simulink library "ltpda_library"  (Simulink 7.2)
settings: Solver=ode45  SolverMode=SingleTasking  StartTime=0.0  StopTime=10.0  RelTol=1e-3
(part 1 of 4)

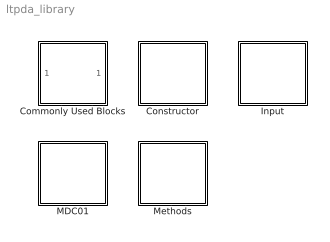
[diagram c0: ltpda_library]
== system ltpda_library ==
  Commonly Used Blocks : Subsystem
  Constructor : Subsystem  Tag=subsystem  AncestorBlock=libraryBase/SubSystName
  Input : Subsystem
  MDC01 : Subsystem  Tag=subsystem  AncestorBlock=libraryBase/SubSystName
  Methods : Subsystem  Tag=subsystem  AncestorBlock=libraryBase/SubSystName

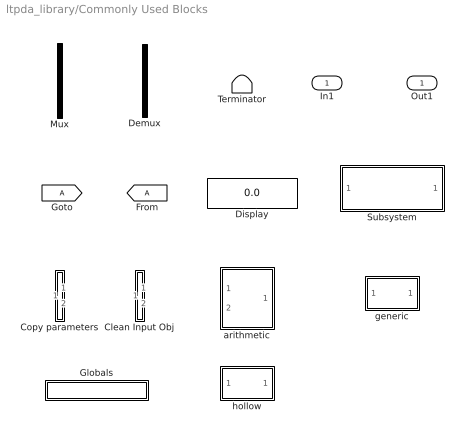
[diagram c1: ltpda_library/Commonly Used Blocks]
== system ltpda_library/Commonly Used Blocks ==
  In1 : Inport  OutDataType=sfix(16)  OutScaling=2^0
  Clean Input Obj : Subsystem
  Copy parameters : Subsystem
  Demux : Demux  Tag=demux  Outputs=2
  Display : Display
  Globals : Subsystem  Tag=globals
  Mux : Mux  Tag=mux  Inputs=2
  Subsystem : Subsystem
  Terminator : Terminator
  arithmetic : Subsystem  Tag=arithmetic
  generic : Subsystem  Tag=function
  hollow : Subsystem  Tag=method ao
  Out1 : Outport  OutDataType=sfix(16)  OutScaling=2^0

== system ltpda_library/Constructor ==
  ltpda_getAOsInTimeSpan : Subsystem  Tag=function  AncestorBlock=libraryBase/function

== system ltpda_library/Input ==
  Constructor : Subsystem  Tag=method ltpda_gui
  Object from list : Subsystem  Tag=input

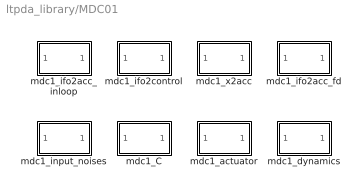
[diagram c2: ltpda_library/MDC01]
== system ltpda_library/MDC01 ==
  mdc1_C : Subsystem  Tag=function  AncestorBlock=libraryBase/function
  mdc1_actuator : Subsystem  Tag=function  AncestorBlock=libraryBase/function
  mdc1_dynamics : Subsystem  Tag=function  AncestorBlock=libraryBase/function
  mdc1_ifo2acc_fd : Subsystem  Tag=function  AncestorBlock=libraryBase/function
  mdc1_ifo2acc_inloop : Subsystem  Tag=function  AncestorBlock=libraryBase/function
  mdc1_ifo2control : Subsystem  Tag=function  AncestorBlock=libraryBase/function
  mdc1_input_noises : Subsystem  Tag=function  AncestorBlock=libraryBase/function
  mdc1_x2acc : Subsystem  Tag=function  AncestorBlock=libraryBase/function

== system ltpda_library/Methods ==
  ao : Subsystem  Tag=subsystem  AncestorBlock=libraryBase/SubSystName

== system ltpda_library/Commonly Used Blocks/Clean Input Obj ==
  In1 : Inport  OutDataType=sfix(16)  OutScaling=2^0
  In2 : Inport  Port=2  OutDataType=sfix(16)  OutScaling=2^0
  cleaninput : M-S-Function  FunctionName=g_cleaninput
  Out1 : Outport  OutDataType=sfix(16)  OutScaling=2^0
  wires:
  In2/1 -> cleaninput/2
  In1/1 -> cleaninput/1
  cleaninput/1 -> Out1/1

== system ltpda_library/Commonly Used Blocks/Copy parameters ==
  In1 : Inport  OutDataType=sfix(16)  OutScaling=2^0
  In2 : Inport  Port=2  OutDataType=sfix(16)  OutScaling=2^0
  copyparam : M-S-Function  FunctionName=g_copyparams
  Out1 : Outport  OutDataType=sfix(16)  OutScaling=2^0
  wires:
  copyparam/1 -> Out1/1
  In1/1 -> copyparam/1
  In2/1 -> copyparam/2

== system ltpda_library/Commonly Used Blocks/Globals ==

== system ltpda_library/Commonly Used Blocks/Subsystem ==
  In1 : Inport  OutDataType=sfix(16)  OutScaling=2^0
  Out1 : Outport  OutDataType=sfix(16)  OutScaling=2^0

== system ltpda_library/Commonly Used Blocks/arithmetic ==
  alpha : Inport  Tag=1  OutDataType=sfix(16)  OutScaling=2^0
  beta : Inport  Tag=2  Port=2  OutDataType=sfix(16)  OutScaling=2^0
  Mux : Mux  Tag=mux  Inputs=2
  arithmetic_func : M-S-Function  Tag=arithmetic  FunctionName=ltpdasim
  Out1 : Outport  OutDataType=sfix(16)  OutScaling=2^0
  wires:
  arithmetic_func/1 -> Out1/1
  Mux/1 -> arithmetic_func/1
  alpha/1 -> Mux/1
  beta/1 -> Mux/2

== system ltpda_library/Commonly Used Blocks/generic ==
  In1 : Inport  OutDataType=sfix(16)  OutScaling=2^0
  generic : M-S-Function  Tag=generic  FunctionName=ltpdasim
  Out1 : Outport  OutDataType=sfix(16)  OutScaling=2^0
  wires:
  generic/1 -> Out1/1
  In1/1 -> generic/1

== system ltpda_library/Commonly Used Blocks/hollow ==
  In1 : Inport  OutDataType=sfix(16)  OutScaling=2^0
  hollow : M-S-Function  FunctionName=ltpdasim
  Out1 : Outport  OutDataType=sfix(16)  OutScaling=2^0
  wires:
  In1/1 -> hollow/1
  hollow/1 -> Out1/1

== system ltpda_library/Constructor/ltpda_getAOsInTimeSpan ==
  In1 : Inport  OutDataType=sfix(16)  OutScaling=2^0
  ltpda_getAOsInTimeSpan : M-S-Function  Tag=ltpda_getAOsInTimeSpan  FunctionName=ltpdasim
  Out1 : Outport  OutDataType=sfix(16)  OutScaling=2^0
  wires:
  In1/1 -> ltpda_getAOsInTimeSpan/1
  ltpda_getAOsInTimeSpan/1 -> Out1/1

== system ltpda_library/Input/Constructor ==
  Ground : Ground
  g_constructor : M-S-Function  Tag=g_constructor  FunctionName=ltpdasim
  Out1 : Outport  OutDataType=sfix(16)  OutScaling=2^0
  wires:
  g_constructor/1 -> Out1/1
  Ground/1 -> g_constructor/1

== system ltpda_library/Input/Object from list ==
  Input : Constant  Value=0  OutDataType=sfix(16)  OutScaling=2^0
  Input AO : Outport  OutDataType=sfix(16)  OutScaling=2^0
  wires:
  Input/1 -> Input AO/1

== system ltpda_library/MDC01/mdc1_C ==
  In1 : Inport  OutDataType=sfix(16)  OutScaling=2^0
  ltpda_mdc1_C : M-S-Function  Tag=ltpda_mdc1_C  FunctionName=ltpdasim
  Out1 : Outport  OutDataType=sfix(16)  OutScaling=2^0
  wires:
  In1/1 -> ltpda_mdc1_C/1
  ltpda_mdc1_C/1 -> Out1/1

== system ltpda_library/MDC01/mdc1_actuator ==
  In1 : Inport  OutDataType=sfix(16)  OutScaling=2^0
  ltpda_mdc1_actuator : M-S-Function  Tag=ltpda_mdc1_actuator  FunctionName=ltpdasim
  Out1 : Outport  OutDataType=sfix(16)  OutScaling=2^0
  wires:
  In1/1 -> ltpda_mdc1_actuator/1
  ltpda_mdc1_actuator/1 -> Out1/1

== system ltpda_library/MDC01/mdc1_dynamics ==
  In1 : Inport  OutDataType=sfix(16)  OutScaling=2^0
  ltpda_mdc1_dynamics : M-S-Function  Tag=ltpda_mdc1_dynamics  FunctionName=ltpdasim
  Out1 : Outport  OutDataType=sfix(16)  OutScaling=2^0
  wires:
  In1/1 -> ltpda_mdc1_dynamics/1
  ltpda_mdc1_dynamics/1 -> Out1/1

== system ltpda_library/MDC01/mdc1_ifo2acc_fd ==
  In1 : Inport  OutDataType=sfix(16)  OutScaling=2^0
  ltpda_mdc1_ifo2acc_fd : M-S-Function  Tag=ltpda_mdc1_ifo2acc_fd  FunctionName=ltpdasim
  Out1 : Outport  OutDataType=sfix(16)  OutScaling=2^0
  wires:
  In1/1 -> ltpda_mdc1_ifo2acc_fd/1
  ltpda_mdc1_ifo2acc_fd/1 -> Out1/1

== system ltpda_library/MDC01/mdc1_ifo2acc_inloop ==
  In1 : Inport  OutDataType=sfix(16)  OutScaling=2^0
  ltpda_mdc1_ifo2acc_inloop : M-S-Function  Tag=ltpda_mdc1_ifo2acc_inloop  FunctionName=ltpdasim
  Out1 : Outport  OutDataType=sfix(16)  OutScaling=2^0
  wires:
  In1/1 -> ltpda_mdc1_ifo2acc_inloop/1
  ltpda_mdc1_ifo2acc_inloop/1 -> Out1/1

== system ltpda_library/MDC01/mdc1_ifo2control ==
  In1 : Inport  OutDataType=sfix(16)  OutScaling=2^0
  ltpda_mdc1_ifo2control : M-S-Function  Tag=ltpda_mdc1_ifo2control  FunctionName=ltpdasim
  Out1 : Outport  OutDataType=sfix(16)  OutScaling=2^0
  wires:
  In1/1 -> ltpda_mdc1_ifo2control/1
  ltpda_mdc1_ifo2control/1 -> Out1/1

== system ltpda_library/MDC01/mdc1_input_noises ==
  In1 : Inport  OutDataType=sfix(16)  OutScaling=2^0
  ltpda_mdc1_input_noises : M-S-Function  Tag=ltpda_mdc1_input_noises  FunctionName=ltpdasim
  Out1 : Outport  OutDataType=sfix(16)  OutScaling=2^0
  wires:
  In1/1 -> ltpda_mdc1_input_noises/1
  ltpda_mdc1_input_noises/1 -> Out1/1

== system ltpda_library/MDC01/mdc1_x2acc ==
  In1 : Inport  OutDataType=sfix(16)  OutScaling=2^0
  ltpda_mdc1_x2acc : M-S-Function  Tag=ltpda_mdc1_x2acc  FunctionName=ltpdasim
  Out1 : Outport  OutDataType=sfix(16)  OutScaling=2^0
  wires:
  In1/1 -> ltpda_mdc1_x2acc/1
  ltpda_mdc1_x2acc/1 -> Out1/1

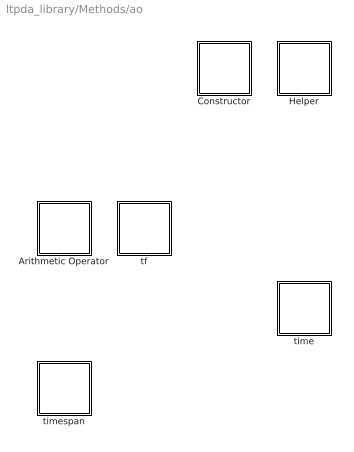
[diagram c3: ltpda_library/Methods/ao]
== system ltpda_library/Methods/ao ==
  Arithmetic Operator : Subsystem  Tag=subsystem  AncestorBlock=libraryBase/SubSystName
  Constructor : Subsystem  Tag=subsystem  AncestorBlock=libraryBase/SubSystName
  Helper : Subsystem  Tag=subsystem  AncestorBlock=libraryBase/SubSystName
  time : Subsystem  Tag=subsystem  AncestorBlock=libraryBase/SubSystName
  tf : Subsystem  Tag=subsystem  AncestorBlock=libraryBase/SubSystName
  time : Subsystem  Tag=subsystem  AncestorBlock=libraryBase/SubSystName
  timespan : Subsystem  Tag=subsystem  AncestorBlock=libraryBase/SubSystName

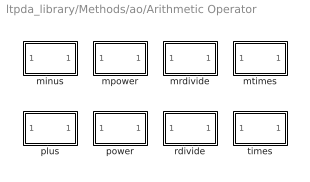
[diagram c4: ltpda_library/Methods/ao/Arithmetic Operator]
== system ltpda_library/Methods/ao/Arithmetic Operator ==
  minus : Subsystem  Tag=method ao  AncestorBlock=libraryBase/function
  mpower : Subsystem  Tag=method ao  AncestorBlock=libraryBase/function
  mrdivide : Subsystem  Tag=method ao  AncestorBlock=libraryBase/function
  mtimes : Subsystem  Tag=method ao  AncestorBlock=libraryBase/function
  plus : Subsystem  Tag=method ao  AncestorBlock=libraryBase/function
  power : Subsystem  Tag=method ao  AncestorBlock=libraryBase/function
  rdivide : Subsystem  Tag=method ao  AncestorBlock=libraryBase/function
  times : Subsystem  Tag=method ao  AncestorBlock=libraryBase/function

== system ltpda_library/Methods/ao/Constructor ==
  ao : Subsystem  Tag=method ao  AncestorBlock=libraryBase/constructor  AncestorBlock=libraryBase/constructor
  rebuild : Subsystem  Tag=method ao  AncestorBlock=libraryBase/constructor

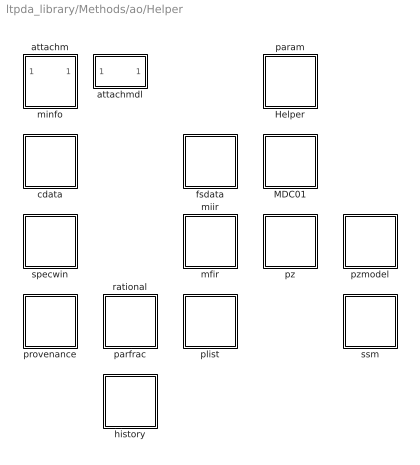
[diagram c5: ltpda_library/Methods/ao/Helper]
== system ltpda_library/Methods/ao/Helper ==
  attachm : Subsystem  Tag=method ao  AncestorBlock=libraryBase/function  AncestorBlock=libraryBase/constructor
  attachmdl : Subsystem  Tag=method ao  AncestorBlock=libraryBase/function
  Helper : Subsystem  Tag=subsystem  AncestorBlock=libraryBase/SubSystName
  MDC01 : Subsystem  Tag=subsystem  AncestorBlock=libraryBase/SubSystName
  cdata : Subsystem  Tag=subsystem  AncestorBlock=libraryBase/SubSystName
  fsdata : Subsystem  Tag=subsystem  AncestorBlock=libraryBase/SubSystName
  history : Subsystem  Tag=subsystem  AncestorBlock=libraryBase/SubSystName
  mfir : Subsystem  Tag=subsystem  AncestorBlock=libraryBase/SubSystName
  miir : Subsystem  Tag=subsystem  AncestorBlock=libraryBase/SubSystName
  miir : Subsystem  Tag=subsystem  AncestorBlock=libraryBase/SubSystName
  minfo : Subsystem  Tag=subsystem  AncestorBlock=libraryBase/SubSystName
  param : Subsystem  Tag=subsystem  AncestorBlock=libraryBase/SubSystName
  plist : Subsystem  Tag=subsystem  AncestorBlock=libraryBase/SubSystName
  provenance : Subsystem  Tag=subsystem  AncestorBlock=libraryBase/SubSystName
  pz : Subsystem  Tag=subsystem  AncestorBlock=libraryBase/SubSystName
  pzmodel : Subsystem  Tag=subsystem  AncestorBlock=libraryBase/SubSystName
  specwin : Subsystem  Tag=subsystem  AncestorBlock=libraryBase/SubSystName
  cdata : Subsystem  Tag=subsystem  AncestorBlock=libraryBase/SubSystName
  fsdata : Subsystem  Tag=subsystem  AncestorBlock=libraryBase/SubSystName
  history : Subsystem  Tag=subsystem  AncestorBlock=libraryBase/SubSystName
  mfir : Subsystem  Tag=subsystem  AncestorBlock=libraryBase/SubSystName
  miir : Subsystem  Tag=subsystem  AncestorBlock=libraryBase/SubSystName
  minfo : Subsystem  Tag=subsystem  AncestorBlock=libraryBase/SubSystName
  param : Subsystem  Tag=subsystem  AncestorBlock=libraryBase/SubSystName
  parfrac : Subsystem  Tag=subsystem  AncestorBlock=libraryBase/SubSystName
  plist : Subsystem  Tag=subsystem  AncestorBlock=libraryBase/SubSystName
  provenance : Subsystem  Tag=subsystem  AncestorBlock=libraryBase/SubSystName
  pz : Subsystem  Tag=subsystem  AncestorBlock=libraryBase/SubSystName
  pzmodel : Subsystem  Tag=subsystem  AncestorBlock=libraryBase/SubSystName
  rational : Subsystem  Tag=subsystem  AncestorBlock=libraryBase/SubSystName
  specwin : Subsystem  Tag=subsystem  AncestorBlock=libraryBase/SubSystName
  ssm : Subsystem  Tag=subsystem  AncestorBlock=libraryBase/SubSystName
  ssm : Subsystem  Tag=subsystem  AncestorBlock=libraryBase/SubSystName

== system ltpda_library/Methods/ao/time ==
  Arithmetic Operator : Subsystem  Tag=subsystem  AncestorBlock=libraryBase/SubSystName

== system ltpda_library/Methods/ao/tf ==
  Constructor : Subsystem  Tag=subsystem  AncestorBlock=libraryBase/SubSystName
  Helper : Subsystem  Tag=subsystem  AncestorBlock=libraryBase/SubSystName
  Output : Subsystem  Tag=subsystem  AncestorBlock=libraryBase/SubSystName
  Relational Operator : Subsystem  Tag=subsystem  AncestorBlock=libraryBase/SubSystName

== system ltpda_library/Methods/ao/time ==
  Arithmetic Operator : Subsystem  Tag=subsystem  AncestorBlock=libraryBase/SubSystName
  Constructor : Subsystem  Tag=subsystem  AncestorBlock=libraryBase/SubSystName
  Helper : Subsystem  Tag=subsystem  AncestorBlock=libraryBase/SubSystName
  Output : Subsystem  Tag=subsystem  AncestorBlock=libraryBase/SubSystName
  Relational Operator : Subsystem  Tag=subsystem  AncestorBlock=libraryBase/SubSystName
  Relational Operator : Subsystem  Tag=subsystem  AncestorBlock=libraryBase/SubSystName

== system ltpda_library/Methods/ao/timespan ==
  Constructor : Subsystem  Tag=subsystem  AncestorBlock=libraryBase/SubSystName
  Helper : Subsystem  Tag=subsystem  AncestorBlock=libraryBase/SubSystName

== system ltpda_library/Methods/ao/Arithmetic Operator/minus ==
  In1 : Inport  OutDataType=sfix(16)  OutScaling=2^0
  minus : M-S-Function  Tag=minus  FunctionName=ltpdasim
  Out1 : Outport  OutDataType=sfix(16)  OutScaling=2^0
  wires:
  In1/1 -> minus/1
  minus/1 -> Out1/1

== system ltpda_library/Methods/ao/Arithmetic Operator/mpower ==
  In1 : Inport  OutDataType=sfix(16)  OutScaling=2^0
  mpower : M-S-Function  Tag=mpower  FunctionName=ltpdasim
  Out1 : Outport  OutDataType=sfix(16)  OutScaling=2^0
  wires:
  In1/1 -> mpower/1
  mpower/1 -> Out1/1

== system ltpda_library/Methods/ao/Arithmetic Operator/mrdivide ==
  In1 : Inport  OutDataType=sfix(16)  OutScaling=2^0
  mrdivide : M-S-Function  Tag=mrdivide  FunctionName=ltpdasim
  Out1 : Outport  OutDataType=sfix(16)  OutScaling=2^0
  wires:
  In1/1 -> mrdivide/1
  mrdivide/1 -> Out1/1

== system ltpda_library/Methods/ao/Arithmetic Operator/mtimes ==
  In1 : Inport  OutDataType=sfix(16)  OutScaling=2^0
  mtimes : M-S-Function  Tag=mtimes  FunctionName=ltpdasim
  Out1 : Outport  OutDataType=sfix(16)  OutScaling=2^0
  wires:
  In1/1 -> mtimes/1
  mtimes/1 -> Out1/1

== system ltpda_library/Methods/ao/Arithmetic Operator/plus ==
  In1 : Inport  OutDataType=sfix(16)  OutScaling=2^0
  plus : M-S-Function  Tag=plus  FunctionName=ltpdasim
  Out1 : Outport  OutDataType=sfix(16)  OutScaling=2^0
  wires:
  In1/1 -> plus/1
  plus/1 -> Out1/1

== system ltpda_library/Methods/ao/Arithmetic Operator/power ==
  In1 : Inport  OutDataType=sfix(16)  OutScaling=2^0
  power : M-S-Function  Tag=power  FunctionName=ltpdasim
  Out1 : Outport  OutDataType=sfix(16)  OutScaling=2^0
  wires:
  In1/1 -> power/1
  power/1 -> Out1/1

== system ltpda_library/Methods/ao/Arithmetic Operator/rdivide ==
  In1 : Inport  OutDataType=sfix(16)  OutScaling=2^0
  rdivide : M-S-Function  Tag=rdivide  FunctionName=ltpdasim
  Out1 : Outport  OutDataType=sfix(16)  OutScaling=2^0
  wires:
  In1/1 -> rdivide/1
  rdivide/1 -> Out1/1

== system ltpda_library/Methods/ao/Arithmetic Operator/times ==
  In1 : Inport  OutDataType=sfix(16)  OutScaling=2^0
  times : M-S-Function  Tag=times  FunctionName=ltpdasim
  Out1 : Outport  OutDataType=sfix(16)  OutScaling=2^0
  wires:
  In1/1 -> times/1
  times/1 -> Out1/1

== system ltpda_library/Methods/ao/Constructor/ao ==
  Ground : Ground
  ao : M-S-Function  Tag=ao  FunctionName=ltpdasim
  Out1 : Outport  OutDataType=sfix(16)  OutScaling=2^0
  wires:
  Ground/1 -> ao/1
  ao/1 -> Out1/1

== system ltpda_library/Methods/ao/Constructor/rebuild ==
  Ground : Ground
  rebuild : M-S-Function  Tag=rebuild  FunctionName=ltpdasim
  Out1 : Outport  OutDataType=sfix(16)  OutScaling=2^0
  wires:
  Ground/1 -> rebuild/1
  rebuild/1 -> Out1/1

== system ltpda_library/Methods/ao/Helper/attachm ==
  In1 : Inport  OutDataType=sfix(16)  OutScaling=2^0
  rebuild : M-S-Function  Tag=attachm  Tag=rebuild  FunctionName=ltpdasim
  Out1 : Outport  OutDataType=sfix(16)  OutScaling=2^0
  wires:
  In1/1 -> rebuild/1
  rebuild/1 -> Out1/1

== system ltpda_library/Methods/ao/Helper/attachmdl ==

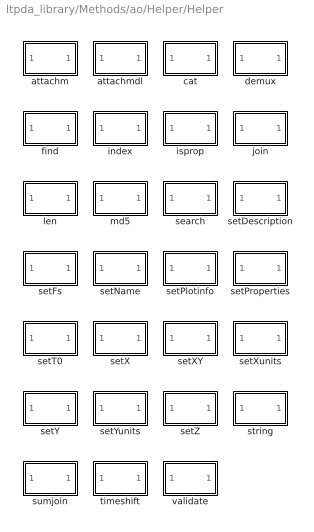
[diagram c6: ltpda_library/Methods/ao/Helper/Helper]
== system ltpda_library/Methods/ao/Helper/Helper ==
  attachm : Subsystem  Tag=method ao  AncestorBlock=libraryBase/function
  attachmdl : Subsystem  Tag=method ao  AncestorBlock=libraryBase/function
  cat : Subsystem  Tag=method ao  AncestorBlock=libraryBase/function
  demux : Subsystem  Tag=method ao  AncestorBlock=libraryBase/function
  find : Subsystem  Tag=method ao  AncestorBlock=libraryBase/function
  index : Subsystem  Tag=method ao  AncestorBlock=libraryBase/function
  isprop : Subsystem  Tag=method ao  AncestorBlock=libraryBase/function
  join : Subsystem  Tag=method ao  AncestorBlock=libraryBase/function
  len : Subsystem  Tag=method ao  AncestorBlock=libraryBase/function
  md5 : Subsystem  Tag=method ao  AncestorBlock=libraryBase/function
  search : Subsystem  Tag=method ao  AncestorBlock=libraryBase/function
  setDescription : Subsystem  Tag=method ao  AncestorBlock=libraryBase/function
  setFs : Subsystem  Tag=method ao  AncestorBlock=libraryBase/function
  setName : Subsystem  Tag=method ao  AncestorBlock=libraryBase/function
  setPlotinfo : Subsystem  Tag=method ao  AncestorBlock=libraryBase/function
  setProperties : Subsystem  Tag=method ao  AncestorBlock=libraryBase/function
  setPlotinfo : Subsystem  Tag=method ao  AncestorBlock=libraryBase/function
  setProperties : Subsystem  Tag=method ao  AncestorBlock=libraryBase/function
  setT0 : Subsystem  Tag=method ao  AncestorBlock=libraryBase/function
  setX : Subsystem  Tag=method ao  AncestorBlock=libraryBase/function
  setXY : Subsystem  Tag=method ao  AncestorBlock=libraryBase/function
  setXunits : Subsystem  Tag=method ao  AncestorBlock=libraryBase/function
  setY : Subsystem  Tag=method ao  AncestorBlock=libraryBase/function
  setYunits : Subsystem  Tag=method ao  AncestorBlock=libraryBase/function
  setZ : Subsystem  Tag=method ao  AncestorBlock=libraryBase/function
  string : Subsystem  Tag=method ao  AncestorBlock=libraryBase/function
  sumjoin : Subsystem  Tag=method ao  AncestorBlock=libraryBase/function
  sumjoin : Subsystem  Tag=method ao  AncestorBlock=libraryBase/function
  timeshift : Subsystem  Tag=method ao  AncestorBlock=libraryBase/function
  validate : Subsystem  Tag=method ao  AncestorBlock=libraryBase/function

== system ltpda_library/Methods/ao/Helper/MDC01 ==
  mdc1_ifo2acc_fd : Subsystem  Tag=method ao  AncestorBlock=libraryBase/function
  mdc1_ifo2acc_inloop : Subsystem  Tag=method ao  AncestorBlock=libraryBase/function
  mdc1_ifo2control : Subsystem  Tag=method ao  AncestorBlock=libraryBase/function

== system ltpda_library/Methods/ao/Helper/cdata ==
  Constructor : Subsystem  Tag=subsystem  AncestorBlock=libraryBase/SubSystName
  Helper : Subsystem  Tag=subsystem  AncestorBlock=libraryBase/SubSystName
  Output : Subsystem  Tag=subsystem  AncestorBlock=libraryBase/SubSystName
  Relational Operator : Subsystem  Tag=subsystem  AncestorBlock=libraryBase/SubSystName

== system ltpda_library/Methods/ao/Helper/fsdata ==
  Constructor : Subsystem  Tag=subsystem  AncestorBlock=libraryBase/SubSystName
  Helper : Subsystem  Tag=subsystem  AncestorBlock=libraryBase/SubSystName
  Output : Subsystem  Tag=subsystem  AncestorBlock=libraryBase/SubSystName
  Relational Operator : Subsystem  Tag=subsystem  AncestorBlock=libraryBase/SubSystName

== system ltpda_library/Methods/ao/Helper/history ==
  Constructor : Subsystem  Tag=subsystem  AncestorBlock=libraryBase/SubSystName
  Helper : Subsystem  Tag=subsystem  AncestorBlock=libraryBase/SubSystName
  Output : Subsystem  Tag=subsystem  AncestorBlock=libraryBase/SubSystName
  Relational Operator : Subsystem  Tag=subsystem  AncestorBlock=libraryBase/SubSystName

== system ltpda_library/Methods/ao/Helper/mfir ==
  Constructor : Subsystem  Tag=subsystem  AncestorBlock=libraryBase/SubSystName
  Helper : Subsystem  Tag=subsystem  AncestorBlock=libraryBase/SubSystName
  Output : Subsystem  Tag=subsystem  AncestorBlock=libraryBase/SubSystName
  Relational Operator : Subsystem  Tag=subsystem  AncestorBlock=libraryBase/SubSystName
  Signal Processing : Subsystem  Tag=subsystem  AncestorBlock=libraryBase/SubSystName
  Statespace : Subsystem  Tag=subsystem  AncestorBlock=libraryBase/SubSystName

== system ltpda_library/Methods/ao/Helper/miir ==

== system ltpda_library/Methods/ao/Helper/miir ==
  Constructor : Subsystem  Tag=subsystem  AncestorBlock=libraryBase/SubSystName
  Helper : Subsystem  Tag=subsystem  AncestorBlock=libraryBase/SubSystName
  Output : Subsystem  Tag=subsystem  AncestorBlock=libraryBase/SubSystName
  Relational Operator : Subsystem  Tag=subsystem  AncestorBlock=libraryBase/SubSystName
  Signal Processing : Subsystem  Tag=subsystem  AncestorBlock=libraryBase/SubSystName
  Statespace : Subsystem  Tag=subsystem  AncestorBlock=libraryBase/SubSystName

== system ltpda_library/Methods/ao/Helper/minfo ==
  Constructor : Subsystem  Tag=subsystem  AncestorBlock=libraryBase/SubSystName
  Helper : Subsystem  Tag=subsystem  AncestorBlock=libraryBase/SubSystName
  Output : Subsystem  Tag=subsystem  AncestorBlock=libraryBase/SubSystName
  Relational Operator : Subsystem  Tag=subsystem  AncestorBlock=libraryBase/SubSystName

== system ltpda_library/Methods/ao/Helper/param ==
  Constructor : Subsystem  Tag=subsystem  AncestorBlock=libraryBase/SubSystName
  Helper : Subsystem  Tag=subsystem  AncestorBlock=libraryBase/SubSystName
  Output : Subsystem  Tag=subsystem  AncestorBlock=libraryBase/SubSystName
  Relational Operator : Subsystem  Tag=subsystem  AncestorBlock=libraryBase/SubSystName

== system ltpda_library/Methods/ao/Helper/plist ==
  Constructor : Subsystem  Tag=subsystem  AncestorBlock=libraryBase/SubSystName
  Helper : Subsystem  Tag=subsystem  AncestorBlock=libraryBase/SubSystName
  Output : Subsystem  Tag=subsystem  AncestorBlock=libraryBase/SubSystName
  Relational Operator : Subsystem  Tag=subsystem  AncestorBlock=libraryBase/SubSystName
  Signal Processing : Subsystem  Tag=subsystem  AncestorBlock=libraryBase/SubSystName

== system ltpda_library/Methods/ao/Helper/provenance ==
  Constructor : Subsystem  Tag=subsystem  AncestorBlock=libraryBase/SubSystName
  Helper : Subsystem  Tag=subsystem  AncestorBlock=libraryBase/SubSystName
  Output : Subsystem  Tag=subsystem  AncestorBlock=libraryBase/SubSystName
  Relational Operator : Subsystem  Tag=subsystem  AncestorBlock=libraryBase/SubSystName

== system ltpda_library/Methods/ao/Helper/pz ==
  Constructor : Subsystem  Tag=subsystem  AncestorBlock=libraryBase/SubSystName
  Helper : Subsystem  Tag=subsystem  AncestorBlock=libraryBase/SubSystName
  Output : Subsystem  Tag=subsystem  AncestorBlock=libraryBase/SubSystName
  Relational Operator : Subsystem  Tag=subsystem  AncestorBlock=libraryBase/SubSystName
  Signal Processing : Subsystem  Tag=subsystem  AncestorBlock=libraryBase/SubSystName

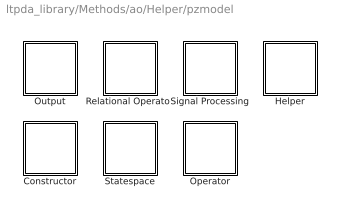
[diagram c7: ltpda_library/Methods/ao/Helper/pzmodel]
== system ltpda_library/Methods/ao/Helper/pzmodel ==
  Constructor : Subsystem  Tag=subsystem  AncestorBlock=libraryBase/SubSystName
  Helper : Subsystem  Tag=subsystem  AncestorBlock=libraryBase/SubSystName
  Operator : Subsystem  Tag=subsystem  AncestorBlock=libraryBase/SubSystName
  Output : Subsystem  Tag=subsystem  AncestorBlock=libraryBase/SubSystName
  Relational Operator : Subsystem  Tag=subsystem  AncestorBlock=libraryBase/SubSystName
  Signal Processing : Subsystem  Tag=subsystem  AncestorBlock=libraryBase/SubSystName
  Statespace : Subsystem  Tag=subsystem  AncestorBlock=libraryBase/SubSystName

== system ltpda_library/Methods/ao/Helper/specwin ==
  Constructor : Subsystem  Tag=subsystem  AncestorBlock=libraryBase/SubSystName
  Trigonometry : Subsystem  Tag=subsystem  AncestorBlock=libraryBase/SubSystName

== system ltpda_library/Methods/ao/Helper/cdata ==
  Constructor : Subsystem  Tag=subsystem  AncestorBlock=libraryBase/SubSystName
  Helper : Subsystem  Tag=subsystem  AncestorBlock=libraryBase/SubSystName
  Output : Subsystem  Tag=subsystem  AncestorBlock=libraryBase/SubSystName
  Relational Operator : Subsystem  Tag=subsystem  AncestorBlock=libraryBase/SubSystName

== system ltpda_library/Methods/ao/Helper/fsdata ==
  Constructor : Subsystem  Tag=subsystem  AncestorBlock=libraryBase/SubSystName
  Helper : Subsystem  Tag=subsystem  AncestorBlock=libraryBase/SubSystName
  Output : Subsystem  Tag=subsystem  AncestorBlock=libraryBase/SubSystName
  Relational Operator : Subsystem  Tag=subsystem  AncestorBlock=libraryBase/SubSystName

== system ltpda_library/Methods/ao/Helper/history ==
  Constructor : Subsystem  Tag=subsystem  AncestorBlock=libraryBase/SubSystName
  Helper : Subsystem  Tag=subsystem  AncestorBlock=libraryBase/SubSystName
  Output : Subsystem  Tag=subsystem  AncestorBlock=libraryBase/SubSystName
  Relational Operator : Subsystem  Tag=subsystem  AncestorBlock=libraryBase/SubSystName

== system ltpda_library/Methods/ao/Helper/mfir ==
  Constructor : Subsystem  Tag=subsystem  AncestorBlock=libraryBase/SubSystName
  Helper : Subsystem  Tag=subsystem  AncestorBlock=libraryBase/SubSystName
  Output : Subsystem  Tag=subsystem  AncestorBlock=libraryBase/SubSystName
  Relational Operator : Subsystem  Tag=subsystem  AncestorBlock=libraryBase/SubSystName
  Signal Processing : Subsystem  Tag=subsystem  AncestorBlock=libraryBase/SubSystName

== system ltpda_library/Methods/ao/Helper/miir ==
  Constructor : Subsystem  Tag=subsystem  AncestorBlock=libraryBase/SubSystName
  Helper : Subsystem  Tag=subsystem  AncestorBlock=libraryBase/SubSystName
  Output : Subsystem  Tag=subsystem  AncestorBlock=libraryBase/SubSystName
  Relational Operator : Subsystem  Tag=subsystem  AncestorBlock=libraryBase/SubSystName
  Signal Processing : Subsystem  Tag=subsystem  AncestorBlock=libraryBase/SubSystName

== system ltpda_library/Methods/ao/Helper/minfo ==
  Constructor : Subsystem  Tag=subsystem  AncestorBlock=libraryBase/SubSystName
  Helper : Subsystem  Tag=subsystem  AncestorBlock=libraryBase/SubSystName
  Output : Subsystem  Tag=subsystem  AncestorBlock=libraryBase/SubSystName
  Relational Operator : Subsystem  Tag=subsystem  AncestorBlock=libraryBase/SubSystName

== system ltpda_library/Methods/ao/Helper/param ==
  Constructor : Subsystem  Tag=subsystem  AncestorBlock=libraryBase/SubSystName
  Helper : Subsystem  Tag=subsystem  AncestorBlock=libraryBase/SubSystName
  Output : Subsystem  Tag=subsystem  AncestorBlock=libraryBase/SubSystName
  Relational Operator : Subsystem  Tag=subsystem  AncestorBlock=libraryBase/SubSystName

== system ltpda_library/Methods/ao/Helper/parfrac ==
  Constructor : Subsystem  Tag=subsystem  AncestorBlock=libraryBase/SubSystName
  Helper : Subsystem  Tag=subsystem  AncestorBlock=libraryBase/SubSystName
  Output : Subsystem  Tag=subsystem  AncestorBlock=libraryBase/SubSystName
  Relational Operator : Subsystem  Tag=subsystem  AncestorBlock=libraryBase/SubSystName
  Signal Processing : Subsystem  Tag=subsystem  AncestorBlock=libraryBase/SubSystName

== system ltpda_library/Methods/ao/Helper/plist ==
  Constructor : Subsystem  Tag=subsystem  AncestorBlock=libraryBase/SubSystName
  Helper : Subsystem  Tag=subsystem  AncestorBlock=libraryBase/SubSystName
  Output : Subsystem  Tag=subsystem  AncestorBlock=libraryBase/SubSystName
  Relational Operator : Subsystem  Tag=subsystem  AncestorBlock=libraryBase/SubSystName
  Signal Processing : Subsystem  Tag=subsystem  AncestorBlock=libraryBase/SubSystName

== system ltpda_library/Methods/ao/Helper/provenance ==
  Constructor : Subsystem  Tag=subsystem  AncestorBlock=libraryBase/SubSystName
  Helper : Subsystem  Tag=subsystem  AncestorBlock=libraryBase/SubSystName
  Output : Subsystem  Tag=subsystem  AncestorBlock=libraryBase/SubSystName
  Relational Operator : Subsystem  Tag=subsystem  AncestorBlock=libraryBase/SubSystName

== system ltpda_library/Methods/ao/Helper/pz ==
  Constructor : Subsystem  Tag=subsystem  AncestorBlock=libraryBase/SubSystName
  Helper : Subsystem  Tag=subsystem  AncestorBlock=libraryBase/SubSystName
  Output : Subsystem  Tag=subsystem  AncestorBlock=libraryBase/SubSystName
  Relational Operator : Subsystem  Tag=subsystem  AncestorBlock=libraryBase/SubSystName
  Signal Processing : Subsystem  Tag=subsystem  AncestorBlock=libraryBase/SubSystName

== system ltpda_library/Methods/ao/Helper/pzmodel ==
  Constructor : Subsystem  Tag=subsystem  AncestorBlock=libraryBase/SubSystName
  Helper : Subsystem  Tag=subsystem  AncestorBlock=libraryBase/SubSystName
  Operator : Subsystem  Tag=subsystem  AncestorBlock=libraryBase/SubSystName
  Output : Subsystem  Tag=subsystem  AncestorBlock=libraryBase/SubSystName
  Relational Operator : Subsystem  Tag=subsystem  AncestorBlock=libraryBase/SubSystName
  Signal Processing : Subsystem  Tag=subsystem  AncestorBlock=libraryBase/SubSystName

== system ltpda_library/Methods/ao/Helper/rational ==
  Constructor : Subsystem  Tag=subsystem  AncestorBlock=libraryBase/SubSystName
  Helper : Subsystem  Tag=subsystem  AncestorBlock=libraryBase/SubSystName
  Output : Subsystem  Tag=subsystem  AncestorBlock=libraryBase/SubSystName
  Relational Operator : Subsystem  Tag=subsystem  AncestorBlock=libraryBase/SubSystName
  Helper : Subsystem  Tag=subsystem  AncestorBlock=libraryBase/SubSystName
  Signal Processing : Subsystem  Tag=subsystem  AncestorBlock=libraryBase/SubSystName

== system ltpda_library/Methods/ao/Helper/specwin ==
  Constructor : Subsystem  Tag=subsystem  AncestorBlock=libraryBase/SubSystName
  Helper : Subsystem  Tag=subsystem  AncestorBlock=libraryBase/SubSystName
  Relational Operator : Subsystem  Tag=subsystem  AncestorBlock=libraryBase/SubSystName

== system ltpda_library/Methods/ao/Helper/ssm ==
  Constructor : Subsystem  Tag=subsystem  AncestorBlock=libraryBase/SubSystName

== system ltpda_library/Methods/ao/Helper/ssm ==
  Constructor : Subsystem  Tag=subsystem  AncestorBlock=libraryBase/SubSystName
  Helper : Subsystem  Tag=subsystem  AncestorBlock=libraryBase/SubSystName

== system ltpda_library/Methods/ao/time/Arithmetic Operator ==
  ssm2miir : Subsystem  Tag=method ssm  AncestorBlock=libraryBase/function
  ssm2pzmodel : Subsystem  Tag=method ssm  AncestorBlock=libraryBase/function
  ssm2rational : Subsystem  Tag=method ssm  AncestorBlock=libraryBase/function
  ssm2ss : Subsystem  Tag=method ssm  AncestorBlock=libraryBase/function
  subsparams : Subsystem  Tag=method ssm  AncestorBlock=libraryBase/function

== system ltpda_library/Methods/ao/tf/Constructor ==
  rebuild : Subsystem  Tag=method tf  AncestorBlock=libraryBase/constructor
  tf : Subsystem  Tag=method tf  AncestorBlock=libraryBase/constructor

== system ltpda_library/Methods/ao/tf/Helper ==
  isprop : Subsystem  Tag=method tf  AncestorBlock=libraryBase/function
  setIunits : Subsystem  Tag=method tf  AncestorBlock=libraryBase/function
  setName : Subsystem  Tag=method tf  AncestorBlock=libraryBase/function
  setOunits : Subsystem  Tag=method tf  AncestorBlock=libraryBase/function
  setProperties : Subsystem  Tag=method tf  AncestorBlock=libraryBase/function

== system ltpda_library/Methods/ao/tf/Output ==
  char : Subsystem  Tag=method tf  AncestorBlock=libraryBase/output
  display : Subsystem  Tag=method tf  AncestorBlock=libraryBase/output
  report : Subsystem  Tag=method tf  AncestorBlock=libraryBase/output
  save : Subsystem  Tag=method tf  AncestorBlock=libraryBase/output
  string : Subsystem  Tag=method tf  AncestorBlock=libraryBase/output
  type : Subsystem  Tag=method tf  AncestorBlock=libraryBase/output

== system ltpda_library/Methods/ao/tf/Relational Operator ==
  eq : Subsystem  Tag=method tf  AncestorBlock=libraryBase/function
  ne : Subsystem  Tag=method tf  AncestorBlock=libraryBase/function

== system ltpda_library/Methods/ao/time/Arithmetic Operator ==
  minus : Subsystem  Tag=method time  AncestorBlock=libraryBase/function
  plus : Subsystem  Tag=method time  AncestorBlock=libraryBase/function

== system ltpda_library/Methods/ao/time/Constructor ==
  time : Subsystem  Tag=method time  AncestorBlock=libraryBase/constructor  AncestorBlock=libraryBase/constructor

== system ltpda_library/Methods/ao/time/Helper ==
  getTimezones : Subsystem  Tag=method time  AncestorBlock=libraryBase/function
  isprop : Subsystem  Tag=method time  AncestorBlock=libraryBase/function
  string : Subsystem  Tag=method time  AncestorBlock=libraryBase/function  Tag=method time  AncestorBlock=libraryBase/function

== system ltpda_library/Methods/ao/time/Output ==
  char : Subsystem  Tag=method time  AncestorBlock=libraryBase/output
  display : Subsystem  Tag=method time  AncestorBlock=libraryBase/output
  format : Subsystem  Tag=method time  AncestorBlock=libraryBase/output

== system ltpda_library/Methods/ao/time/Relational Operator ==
  eq : Subsystem  Tag=method time  AncestorBlock=libraryBase/function
  ne : Subsystem  Tag=method time  AncestorBlock=libraryBase/function

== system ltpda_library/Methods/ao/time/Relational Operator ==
  eq : Subsystem  Tag=method time  AncestorBlock=libraryBase/function
  ne : Subsystem  Tag=method time  AncestorBlock=libraryBase/function

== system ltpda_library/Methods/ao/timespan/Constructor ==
  rebuild : Subsystem  Tag=method timespan  AncestorBlock=libraryBase/constructor
  timespan : Subsystem  Tag=method timespan  AncestorBlock=libraryBase/constructor
  timespan : Subsystem  Tag=method timespan  AncestorBlock=libraryBase/constructor

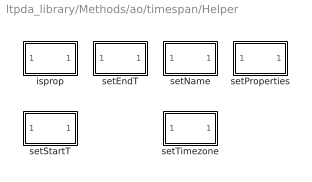
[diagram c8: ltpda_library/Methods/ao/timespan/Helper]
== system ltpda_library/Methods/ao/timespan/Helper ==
  isprop : Subsystem  Tag=method timespan  AncestorBlock=libraryBase/function
  setEndT : Subsystem  Tag=method timespan  AncestorBlock=libraryBase/function
  isprop : Subsystem  Tag=method timespan  AncestorBlock=libraryBase/function  Tag=method timespan  AncestorBlock=libraryBase/function
  setEndT : Subsystem  Tag=method timespan  AncestorBlock=libraryBase/function  Tag=method timespan  AncestorBlock=libraryBase/function
  setName : Subsystem  Tag=method timespan  AncestorBlock=libraryBase/function
  setProperties : Subsystem  Tag=method timespan  AncestorBlock=libraryBase/function  Tag=method timespan  AncestorBlock=libraryBase/function
  setStartT : Subsystem  Tag=method timespan  Tag=method timespan  AncestorBlock=libraryBase/function
  setTimezone : Subsystem  Tag=method timespan  AncestorBlock=libraryBase/function

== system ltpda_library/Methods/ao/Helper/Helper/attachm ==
  In1 : Inport  OutDataType=sfix(16)  OutScaling=2^0
  attachm : M-S-Function  Tag=attachm  FunctionName=ltpdasim
  Out1 : Outport  OutDataType=sfix(16)  OutScaling=2^0
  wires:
  In1/1 -> attachm/1
  attachm/1 -> Out1/1

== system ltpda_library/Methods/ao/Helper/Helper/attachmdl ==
  In1 : Inport  OutDataType=sfix(16)  OutScaling=2^0
  attachmdl : M-S-Function  Tag=attachmdl  FunctionName=ltpdasim
  Out1 : Outport  OutDataType=sfix(16)  OutScaling=2^0
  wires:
  In1/1 -> attachmdl/1
  attachmdl/1 -> Out1/1

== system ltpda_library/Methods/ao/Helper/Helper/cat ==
  In1 : Inport  OutDataType=sfix(16)  OutScaling=2^0
  cat : M-S-Function  Tag=cat  FunctionName=ltpdasim
  Out1 : Outport  OutDataType=sfix(16)  OutScaling=2^0
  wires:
  In1/1 -> cat/1
  cat/1 -> Out1/1

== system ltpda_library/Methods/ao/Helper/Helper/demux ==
  In1 : Inport  OutDataType=sfix(16)  OutScaling=2^0
  demux : M-S-Function  Tag=demux  FunctionName=ltpdasim
  Out1 : Outport  OutDataType=sfix(16)  OutScaling=2^0
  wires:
  In1/1 -> demux/1
  demux/1 -> Out1/1

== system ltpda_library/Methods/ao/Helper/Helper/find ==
  In1 : Inport  OutDataType=sfix(16)  OutScaling=2^0
  find : M-S-Function  Tag=find  FunctionName=ltpdasim
  Out1 : Outport  OutDataType=sfix(16)  OutScaling=2^0
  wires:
  In1/1 -> find/1
  find/1 -> Out1/1

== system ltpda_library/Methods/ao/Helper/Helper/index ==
  In1 : Inport  OutDataType=sfix(16)  OutScaling=2^0
  index : M-S-Function  Tag=index  FunctionName=ltpdasim
  Out1 : Outport  OutDataType=sfix(16)  OutScaling=2^0
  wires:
  In1/1 -> index/1
  index/1 -> Out1/1

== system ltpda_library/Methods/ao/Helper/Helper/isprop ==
  In1 : Inport  OutDataType=sfix(16)  OutScaling=2^0
  isprop : M-S-Function  Tag=isprop  FunctionName=ltpdasim
  Out1 : Outport  OutDataType=sfix(16)  OutScaling=2^0
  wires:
  In1/1 -> isprop/1
  isprop/1 -> Out1/1

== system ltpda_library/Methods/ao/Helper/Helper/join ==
  In1 : Inport  OutDataType=sfix(16)  OutScaling=2^0
  join : M-S-Function  Tag=join  FunctionName=ltpdasim
  Out1 : Outport  OutDataType=sfix(16)  OutScaling=2^0
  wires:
  In1/1 -> join/1
  join/1 -> Out1/1

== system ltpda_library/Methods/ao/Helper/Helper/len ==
  In1 : Inport  OutDataType=sfix(16)  OutScaling=2^0
  len : M-S-Function  Tag=len  FunctionName=ltpdasim
  Out1 : Outport  OutDataType=sfix(16)  OutScaling=2^0
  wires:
  In1/1 -> len/1
  len/1 -> Out1/1

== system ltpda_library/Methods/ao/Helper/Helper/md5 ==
  In1 : Inport  OutDataType=sfix(16)  OutScaling=2^0
  md5 : M-S-Function  Tag=md5  FunctionName=ltpdasim
  Out1 : Outport  OutDataType=sfix(16)  OutScaling=2^0
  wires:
  In1/1 -> md5/1
  md5/1 -> Out1/1

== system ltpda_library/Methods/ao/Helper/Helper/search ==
  In1 : Inport  OutDataType=sfix(16)  OutScaling=2^0
  search : M-S-Function  Tag=search  FunctionName=ltpdasim
  Out1 : Outport  OutDataType=sfix(16)  OutScaling=2^0
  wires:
  In1/1 -> search/1
  search/1 -> Out1/1

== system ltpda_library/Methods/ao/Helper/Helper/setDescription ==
  In1 : Inport  OutDataType=sfix(16)  OutScaling=2^0
  setDescription : M-S-Function  Tag=setDescription  FunctionName=ltpdasim
  Out1 : Outport  OutDataType=sfix(16)  OutScaling=2^0
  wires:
  In1/1 -> setDescription/1
  setDescription/1 -> Out1/1

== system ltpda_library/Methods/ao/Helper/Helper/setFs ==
  In1 : Inport  OutDataType=sfix(16)  OutScaling=2^0
  setFs : M-S-Function  Tag=setFs  FunctionName=ltpdasim
  Out1 : Outport  OutDataType=sfix(16)  OutScaling=2^0
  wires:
  In1/1 -> setFs/1
  setFs/1 -> Out1/1

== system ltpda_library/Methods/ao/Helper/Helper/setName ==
  In1 : Inport  OutDataType=sfix(16)  OutScaling=2^0
  setName : M-S-Function  Tag=setName  FunctionName=ltpdasim
  Out1 : Outport  OutDataType=sfix(16)  OutScaling=2^0
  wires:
  In1/1 -> setName/1
  setName/1 -> Out1/1

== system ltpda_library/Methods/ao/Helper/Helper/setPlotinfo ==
  In1 : Inport  OutDataType=sfix(16)  OutScaling=2^0
  setPlotinfo : M-S-Function  Tag=setPlotinfo  FunctionName=ltpdasim
  Out1 : Outport  OutDataType=sfix(16)  OutScaling=2^0
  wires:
  In1/1 -> setPlotinfo/1
  setPlotinfo/1 -> Out1/1

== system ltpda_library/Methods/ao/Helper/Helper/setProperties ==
  In1 : Inport  OutDataType=sfix(16)  OutScaling=2^0
  setProperties : M-S-Function  Tag=setName  Tag=setProperties  FunctionName=ltpdasim
  Out1 : Outport  OutDataType=sfix(16)  OutScaling=2^0
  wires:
  In1/1 -> setProperties/1
  ?setName/1 -> Out1/1

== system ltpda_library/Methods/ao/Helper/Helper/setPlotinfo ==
  In1 : Inport  OutDataType=sfix(16)  OutScaling=2^0
  setPlotinfo : M-S-Function  Tag=setPlotinfo  FunctionName=ltpdasim
  Out1 : Outport  OutDataType=sfix(16)  OutScaling=2^0
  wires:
  In1/1 -> setPlotinfo/1
  setPlotinfo/1 -> Out1/1

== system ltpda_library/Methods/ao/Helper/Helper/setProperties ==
  In1 : Inport  OutDataType=sfix(16)  OutScaling=2^0
  setProperties : M-S-Function  Tag=setProperties  FunctionName=ltpdasim
  Out1 : Outport  OutDataType=sfix(16)  OutScaling=2^0
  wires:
  In1/1 -> setProperties/1
  setProperties/1 -> Out1/1

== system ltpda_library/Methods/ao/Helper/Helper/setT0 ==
  In1 : Inport  OutDataType=sfix(16)  OutScaling=2^0
  setT0 : M-S-Function  Tag=setT0  FunctionName=ltpdasim
  Out1 : Outport  OutDataType=sfix(16)  OutScaling=2^0
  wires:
  In1/1 -> setT0/1
  setT0/1 -> Out1/1

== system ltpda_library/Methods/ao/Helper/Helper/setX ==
  In1 : Inport  OutDataType=sfix(16)  OutScaling=2^0
  setX : M-S-Function  Tag=setX  FunctionName=ltpdasim
  Out1 : Outport  OutDataType=sfix(16)  OutScaling=2^0
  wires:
  In1/1 -> setX/1
  setX/1 -> Out1/1

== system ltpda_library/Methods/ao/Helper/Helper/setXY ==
  In1 : Inport  OutDataType=sfix(16)  OutScaling=2^0
  setXY : M-S-Function  Tag=setXY  FunctionName=ltpdasim
  Out1 : Outport  OutDataType=sfix(16)  OutScaling=2^0
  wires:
  In1/1 -> setXY/1
  setXY/1 -> Out1/1

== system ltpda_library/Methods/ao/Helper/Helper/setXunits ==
  In1 : Inport  OutDataType=sfix(16)  OutScaling=2^0
  setXunits : M-S-Function  Tag=setXunits  FunctionName=ltpdasim
  Out1 : Outport  OutDataType=sfix(16)  OutScaling=2^0
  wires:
  In1/1 -> setXunits/1
  setXunits/1 -> Out1/1

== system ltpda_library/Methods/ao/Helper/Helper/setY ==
  In1 : Inport  OutDataType=sfix(16)  OutScaling=2^0
  setY : M-S-Function  Tag=setY  FunctionName=ltpdasim
  Out1 : Outport  OutDataType=sfix(16)  OutScaling=2^0
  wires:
  In1/1 -> setY/1
  setY/1 -> Out1/1

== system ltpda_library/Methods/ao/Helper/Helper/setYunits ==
  In1 : Inport  OutDataType=sfix(16)  OutScaling=2^0
  setYunits : M-S-Function  Tag=setYunits  FunctionName=ltpdasim
  Out1 : Outport  OutDataType=sfix(16)  OutScaling=2^0
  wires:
  In1/1 -> setYunits/1
  setYunits/1 -> Out1/1

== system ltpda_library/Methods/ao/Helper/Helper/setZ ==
  In1 : Inport  OutDataType=sfix(16)  OutScaling=2^0
  setZ : M-S-Function  Tag=setZ  FunctionName=ltpdasim
  Out1 : Outport  OutDataType=sfix(16)  OutScaling=2^0
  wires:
  In1/1 -> setZ/1
  setZ/1 -> Out1/1

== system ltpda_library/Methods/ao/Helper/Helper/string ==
  In1 : Inport  OutDataType=sfix(16)  OutScaling=2^0
  string : M-S-Function  Tag=string  FunctionName=ltpdasim
  Out1 : Outport  OutDataType=sfix(16)  OutScaling=2^0
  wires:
  In1/1 -> string/1
  string/1 -> Out1/1

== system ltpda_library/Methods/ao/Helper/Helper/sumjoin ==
  In1 : Inport  OutDataType=sfix(16)  OutScaling=2^0
  sumjoin : M-S-Function  Tag=sumjoin  FunctionName=ltpdasim
  Out1 : Outport  OutDataType=sfix(16)  OutScaling=2^0
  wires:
  In1/1 -> sumjoin/1
  sumjoin/1 -> Out1/1

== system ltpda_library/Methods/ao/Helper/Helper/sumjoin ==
  In1 : Inport  OutDataType=sfix(16)  OutScaling=2^0
  sumjoin : M-S-Function  Tag=sumjoin  FunctionName=ltpdasim
  Out1 : Outport  OutDataType=sfix(16)  OutScaling=2^0
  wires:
  In1/1 -> sumjoin/1
  sumjoin/1 -> Out1/1

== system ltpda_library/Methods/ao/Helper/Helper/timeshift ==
  In1 : Inport  OutDataType=sfix(16)  OutScaling=2^0
  timeshift : M-S-Function  Tag=timeshift  FunctionName=ltpdasim
  Out1 : Outport  OutDataType=sfix(16)  OutScaling=2^0
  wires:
  In1/1 -> timeshift/1
  timeshift/1 -> Out1/1

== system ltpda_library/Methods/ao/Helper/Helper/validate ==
  In1 : Inport  OutDataType=sfix(16)  OutScaling=2^0
  validate : M-S-Function  Tag=validate  FunctionName=ltpdasim
  Out1 : Outport  OutDataType=sfix(16)  OutScaling=2^0
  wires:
  In1/1 -> validate/1
  validate/1 -> Out1/1

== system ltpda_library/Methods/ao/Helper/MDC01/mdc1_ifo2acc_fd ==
  In1 : Inport  OutDataType=sfix(16)  OutScaling=2^0
  mdc1_ifo2acc_fd : M-S-Function  Tag=mdc1_ifo2acc_fd  FunctionName=ltpdasim
  Out1 : Outport  OutDataType=sfix(16)  OutScaling=2^0
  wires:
  In1/1 -> mdc1_ifo2acc_fd/1
  mdc1_ifo2acc_fd/1 -> Out1/1

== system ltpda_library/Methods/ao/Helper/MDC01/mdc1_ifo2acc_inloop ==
  In1 : Inport  OutDataType=sfix(16)  OutScaling=2^0
  mdc1_ifo2acc_inloop : M-S-Function  Tag=mdc1_ifo2acc_inloop  FunctionName=ltpdasim
  Out1 : Outport  OutDataType=sfix(16)  OutScaling=2^0
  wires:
  In1/1 -> mdc1_ifo2acc_inloop/1
  mdc1_ifo2acc_inloop/1 -> Out1/1

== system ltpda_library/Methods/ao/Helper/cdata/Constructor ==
  cdata : Subsystem  Tag=method cdata  AncestorBlock=libraryBase/constructor

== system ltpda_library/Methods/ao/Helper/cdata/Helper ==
  isprop : Subsystem  Tag=method cdata  AncestorBlock=libraryBase/function

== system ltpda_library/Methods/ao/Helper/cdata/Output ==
  display : Subsystem  Tag=method cdata  AncestorBlock=libraryBase/output

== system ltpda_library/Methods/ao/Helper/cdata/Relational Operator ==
  eq : Subsystem  Tag=method cdata  AncestorBlock=libraryBase/function
  ne : Subsystem  Tag=method cdata  AncestorBlock=libraryBase/function

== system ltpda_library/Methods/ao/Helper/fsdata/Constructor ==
  fsdata : Subsystem  Tag=method fsdata  AncestorBlock=libraryBase/constructor

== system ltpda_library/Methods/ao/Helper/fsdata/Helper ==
  isprop : Subsystem  Tag=method fsdata  AncestorBlock=libraryBase/function

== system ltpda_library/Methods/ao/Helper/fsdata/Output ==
  char : Subsystem  Tag=method fsdata  AncestorBlock=libraryBase/output
  display : Subsystem  Tag=method fsdata  AncestorBlock=libraryBase/output

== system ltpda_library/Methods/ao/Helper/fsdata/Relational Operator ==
  eq : Subsystem  Tag=method fsdata  AncestorBlock=libraryBase/function
  ne : Subsystem  Tag=method fsdata  AncestorBlock=libraryBase/function

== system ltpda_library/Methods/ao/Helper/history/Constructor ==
  history : Subsystem  Tag=method history  AncestorBlock=libraryBase/constructor
  rebuild : Subsystem  Tag=method history  AncestorBlock=libraryBase/constructor

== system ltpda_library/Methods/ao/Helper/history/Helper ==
  isprop : Subsystem  Tag=method history  AncestorBlock=libraryBase/function

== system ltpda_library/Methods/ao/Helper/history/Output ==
  char : Subsystem  Tag=method history  AncestorBlock=libraryBase/output
  display : Subsystem  Tag=method history  AncestorBlock=libraryBase/output
  dotview : Subsystem  Tag=method history  AncestorBlock=libraryBase/output
  hist2dot : Subsystem  Tag=method history  AncestorBlock=libraryBase/output
  hist2m : Subsystem  Tag=method history  AncestorBlock=libraryBase/output
  plot : Subsystem  Tag=method history  AncestorBlock=libraryBase/output
  string : Subsystem  Tag=method history  AncestorBlock=libraryBase/output

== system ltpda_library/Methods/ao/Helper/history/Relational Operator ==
  eq : Subsystem  Tag=method history  AncestorBlock=libraryBase/function
  ne : Subsystem  Tag=method history  AncestorBlock=libraryBase/function

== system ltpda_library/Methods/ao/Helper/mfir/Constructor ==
  mfir : Subsystem  Tag=method mfir  AncestorBlock=libraryBase/constructor
  rebuild : Subsystem  Tag=method mfir  AncestorBlock=libraryBase/constructor

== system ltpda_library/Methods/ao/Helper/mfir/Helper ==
  isprop : Subsystem  Tag=method mfir  AncestorBlock=libraryBase/function
  redesign : Subsystem  Tag=method mfir  AncestorBlock=libraryBase/function
  setIunits : Subsystem  Tag=method mfir  AncestorBlock=libraryBase/function
  setName : Subsystem  Tag=method mfir  AncestorBlock=libraryBase/function
  setOunits : Subsystem  Tag=method mfir  AncestorBlock=libraryBase/function
  setProperties : Subsystem  Tag=method mfir  AncestorBlock=libraryBase/function

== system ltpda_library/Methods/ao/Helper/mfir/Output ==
  char : Subsystem  Tag=method mfir  AncestorBlock=libraryBase/output
  display : Subsystem  Tag=method mfir  AncestorBlock=libraryBase/output
  save : Subsystem  Tag=method mfir  AncestorBlock=libraryBase/output
  save : Subsystem  Tag=method mfir  AncestorBlock=libraryBase/output
  string : Subsystem  Tag=method mfir  AncestorBlock=libraryBase/output
  type : Subsystem  Tag=method mfir  AncestorBlock=libraryBase/output

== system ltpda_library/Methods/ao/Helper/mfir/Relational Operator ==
  eq : Subsystem  Tag=method mfir  AncestorBlock=libraryBase/function
  ne : Subsystem  Tag=method mfir  AncestorBlock=libraryBase/function

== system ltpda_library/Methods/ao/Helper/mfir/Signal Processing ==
  oldresp : Subsystem  Tag=method mfir  AncestorBlock=libraryBase/function
  resp : Subsystem  Tag=method mfir  AncestorBlock=libraryBase/function

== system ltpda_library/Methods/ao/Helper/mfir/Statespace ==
  report : Subsystem  Tag=method mfir  AncestorBlock=libraryBase/function

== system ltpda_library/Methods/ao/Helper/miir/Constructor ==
  miir : Subsystem  Tag=method miir  AncestorBlock=libraryBase/constructor
  rebuild : Subsystem  Tag=method miir  AncestorBlock=libraryBase/constructor

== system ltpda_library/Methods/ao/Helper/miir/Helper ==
  isprop : Subsystem  Tag=method miir  AncestorBlock=libraryBase/function
  redesign : Subsystem  Tag=method miir  AncestorBlock=libraryBase/function
  setIunits : Subsystem  Tag=method miir  AncestorBlock=libraryBase/function
  setName : Subsystem  Tag=method miir  AncestorBlock=libraryBase/function
  setOunits : Subsystem  Tag=method miir  AncestorBlock=libraryBase/function
  setProperties : Subsystem  Tag=method miir  AncestorBlock=libraryBase/function

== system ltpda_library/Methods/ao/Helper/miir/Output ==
  char : Subsystem  Tag=method miir  AncestorBlock=libraryBase/output
  display : Subsystem  Tag=method miir  AncestorBlock=libraryBase/output
  save : Subsystem  Tag=method miir  AncestorBlock=libraryBase/output
  save : Subsystem  Tag=method miir  AncestorBlock=libraryBase/output
  string : Subsystem  Tag=method miir  AncestorBlock=libraryBase/output
  type : Subsystem  Tag=method miir  AncestorBlock=libraryBase/output

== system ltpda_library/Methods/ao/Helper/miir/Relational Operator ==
  eq : Subsystem  Tag=method miir  AncestorBlock=libraryBase/function
  ne : Subsystem  Tag=method miir  AncestorBlock=libraryBase/function

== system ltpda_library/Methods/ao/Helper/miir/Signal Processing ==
  oldresp : Subsystem  Tag=method miir  AncestorBlock=libraryBase/function
  resp : Subsystem  Tag=method miir  AncestorBlock=libraryBase/function

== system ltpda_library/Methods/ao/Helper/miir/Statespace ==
  report : Subsystem  Tag=method miir  AncestorBlock=libraryBase/function

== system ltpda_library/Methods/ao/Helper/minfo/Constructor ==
  minfo : Subsystem  Tag=method minfo  AncestorBlock=libraryBase/constructor

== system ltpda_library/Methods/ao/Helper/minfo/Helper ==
  isprop : Subsystem  Tag=method minfo  AncestorBlock=libraryBase/function

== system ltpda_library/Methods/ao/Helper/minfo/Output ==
  char : Subsystem  Tag=method minfo  AncestorBlock=libraryBase/output
  display : Subsystem  Tag=method minfo  AncestorBlock=libraryBase/output
